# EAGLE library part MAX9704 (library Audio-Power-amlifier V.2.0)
The MAX9704 stereo class D audio power amplifiers provide class AB amplifier performance with class D efficiency, conserving board space and eliminating the need for a bulky heatsink. Using a class D architecture, these devices deliver up to 15W while offering up to 78% efficiency. Proprietary and patent-protected modulation and switching schemes render the traditional class D output filter unnecessary.
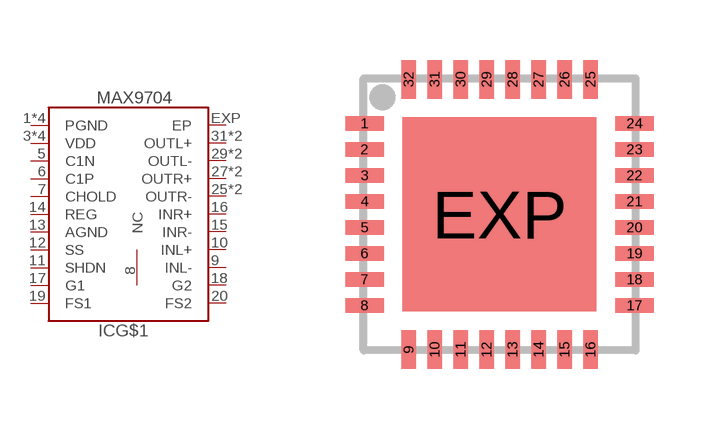
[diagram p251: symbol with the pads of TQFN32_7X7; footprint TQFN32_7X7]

Designator prefix IC; gates G$1=MAX9704 G$2=NC

## MAX9704  [TQFN32_7X7]
1  G$1:PGND  pwr
2  G$1:PGND  pwr
3  G$1:VDD  pwr
4  G$1:VDD  pwr
5  G$1:C1N
6  G$1:C1P
7  G$1:CHOLD
8  G$2:NC  nc
9  G$1:INL-  in
10  G$1:INL+  in
11  G$1:SHDN
12  G$1:SS
13  G$1:AGND  pwr
14  G$1:REG  out
15  G$1:INR-  in
16  G$1:INR+  in
17  G$1:G1  in
18  G$1:G2  in
19  G$1:FS1  in
20  G$1:FS2  in
21  G$1:VDD  pwr
22  G$1:VDD  pwr
23  G$1:PGND  pwr
24  G$1:PGND  pwr
25  G$1:OUTR-  out
26  G$1:OUTR-  out
27  G$1:OUTR+  out
28  G$1:OUTR+  out
29  G$1:OUTL-  out
30  G$1:OUTL-  out
31  G$1:OUTL+  out
32  G$1:OUTL+  out
EXP  G$1:EP  pwr

## Footprint TQFN32_7X7 (pad centres in mm)
TQFN 7x7 mm Source: www.maxim-ic.com/packages .. 90-0125.pdf
smd 0.965 x 0.366: 1 -3.378,2.275; 2 -3.378,1.625; 3 -3.378,0.975; 4 -3.378,0.325; 5 -3.378,-0.325; 6 -3.378,-0.975; 7 -3.378,-1.625; 8 -3.378,-2.275; 17 3.378,-2.275; 18 3.378,-1.625; 19 3.378,-0.975; 20 3.378,-0.325; 21 3.378,0.325; 22 3.378,0.975; 23 3.378,1.625; 24 3.378,2.275
smd 0.366 x 0.965: 9 -2.275,-3.378; 10 -1.625,-3.378; 11 -0.975,-3.378; 12 -0.325,-3.378; 13 0.325,-3.378; 14 0.975,-3.378; 15 1.625,-3.378; 16 2.275,-3.378; 25 2.275,3.378; 26 1.625,3.378; 27 0.975,3.378; 28 0.325,3.378; 29 -0.325,3.378; 30 -0.975,3.378; 31 -1.625,3.378; 32 -2.275,3.378
smd 4.851 x 4.851: EXP 0,0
